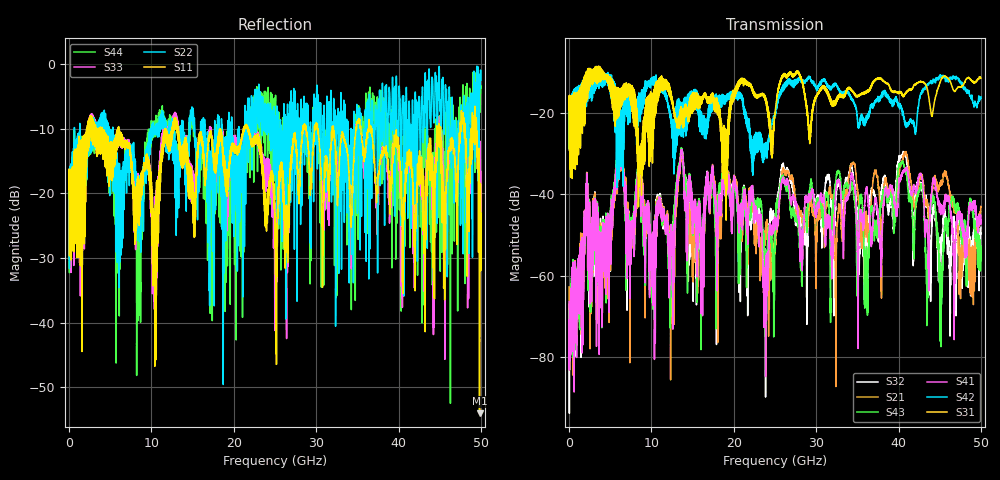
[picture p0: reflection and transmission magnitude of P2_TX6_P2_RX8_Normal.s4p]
!Keysight Technologies,N5225B,MY57041031,A.13.20.10
!Date: Friday, May 31, 2019 11:39:44
!Correction: S11(Full 4 Port(1,2,3,4))
!S12(Full 4 Port(1,2,3,4))
!S13(Full 4 Port(1,2,3,4))
!S14(Full 4 Port(1,2,3,4))
!S21(Full 4 Port(1,2,3,4))
!S22(Full 4 Port(1,2,3,4))
!S23(Full 4 Port(1,2,3,4))
!S24(Full 4 Port(1,2,3,4))
!S31(Full 4 Port(1,2,3,4))
!S32(Full 4 Port(1,2,3,4))
!S33(Full 4 Port(1,2,3,4))
!S34(Full 4 Port(1,2,3,4))
!S41(Full 4 Port(1,2,3,4))
!S42(Full 4 Port(1,2,3,4))
!S43(Full 4 Port(1,2,3,4))
!S44(Full 4 Port(1,2,3,4))
!S4P File: Measurements: <S11,S12,S13,S14>,
!<S21,S22,S23,S24>,
!<S31,S32,S33,S34>,
!<S41,S42,S43,S44>:
# Hz S  dB  R 50.0
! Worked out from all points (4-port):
!   5000 points, 10 MHz to 50 GHz, reference 50 ohm
!   strongest paths, dB at 10 MHz, 12.51 GHz, 25.01 GHz, 37.51 GHz, 50 GHz:
!     S31: -19.3, -16.8, -20.0, -11.6, -11.4
!     S42: -19.5, -21.7, -19.9, -16.3, -16.0
!     S41: -66.4, -54.2, -45.6, -45.5, -46.3
!     S43: -70.8, -60.9, -47.6, -46.5, -52.8
!     S21: -62.8, -51.6, -52.2, -36.8, -43.2
!     S32: -67.0, -57.7, -49.9, -47.3, -48.1
!   lowest |S11| = -54.1 dB at 49.84 GHz (marker M1), VSWR 1.00, Z = 50.2 - j0.109 ohm
!   |S11| at or under -10 dB: 6.028 GHz to 11.67 GHz (5.642 GHz wide, 63.8 % of centre); 21.74 GHz to 28.38 GHz (6.639 GHz wide, 26.5 % of centre); 36.76 GHz to 44.63 GHz (7.869 GHz wide, 19.3 % of centre)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
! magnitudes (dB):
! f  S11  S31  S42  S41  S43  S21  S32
! 10 MHz  -19.4  -19.3  -19.5  -66.4  -70.8  -62.8  -67.0
! 6.23 GHz  -11.3  -15.3  -20.7  -30.9  -30.2  -31.6  -30.7
! 22.13 GHz  -11.6  -13.9  -26.2  -38.0  -39.9  -40.4  -42.6
! 23.82 GHz  -22.8  -16.2  -28.9  -58.8  -64.8  -50.3  -69.3
! 26 GHz  -18.3  -11.0  -13.5  -36.3  -35.8  -34.0  -32.5
! 49.84 GHz  -54.1  -11.1  -16.9  -47.5  -53.9  -47.5  -52.6
! 50 GHz  -23.1  -11.4  -16.0  -46.3  -52.8  -43.2  -48.1
